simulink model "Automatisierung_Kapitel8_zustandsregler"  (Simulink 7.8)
settings: Solver=ode45  StartTime=0.0  StopTime=100  MaxStep=0.2  RelTol=1e-3
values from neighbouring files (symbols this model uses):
  Ac = [0,1,0,0;-1,-1,1,1;0,0,0,1;0.1,0.1,-0.2,-0.2]    [Automatisierung_Kapitel8.m]
  Bc = [bc,bvc]    [Automatisierung_Kapitel8.m]
  Cc = eye(4)    [Automatisierung_Kapitel8.m]
  Dc = [0,0;0,0;0,0;0,0]    [Automatisierung_Kapitel8.m]
  g = 1/((cc+dc*k)*inv(eye(4)-Ad-bd*k)*bd+dc)    [Automatisierung_Kapitel8.m]
  k = -acker(Ad,bd,pd)    [Automatisierung_Kapitel8.m]
  Ta = 2    [Automatisierung_Kapitel8.m]
libraries: simulink x1

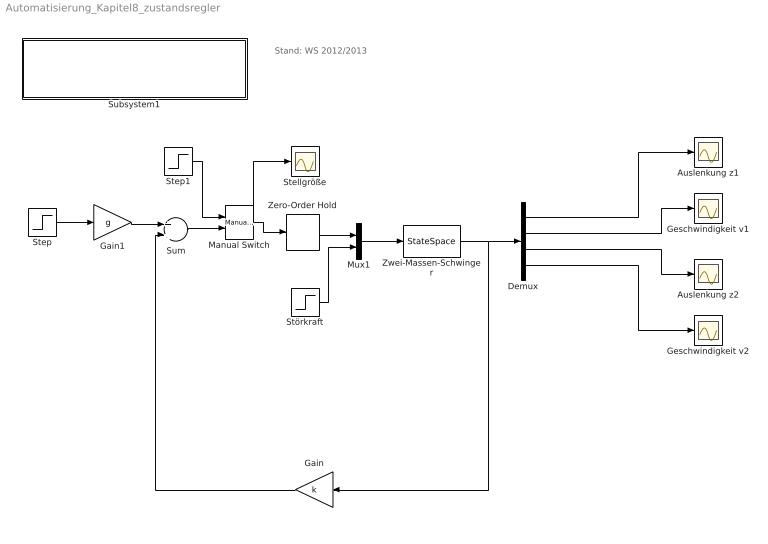
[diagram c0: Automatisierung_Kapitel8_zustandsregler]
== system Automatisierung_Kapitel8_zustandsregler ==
  note: Stand: WS 2012/2013
  Auslenkung z1 : Scope
  Auslenkung z2 : Scope
  Demux : Demux
  Gain : Gain  Gain=k  Multiplication=Matrix(K*u)  SampleTime=Ta
  Gain1 : Gain  Gain=g  SampleTime=Ta
  Geschwindigkeit v1 : Scope
  Geschwindigkeit v2 : Scope
  Manual Switch : simulink/Signal Routing/Manual Switch  sw=0  action=0  varsize=off
  Mux1 : Mux  Inputs=2
  Stellgröße : Scope
  Step : Step  Time=0  SampleTime=Ta
  Step1 : Step  Time=0  SampleTime=0
  Störkraft : Step  Time=20  SampleTime=Ta
  Subsystem1 : Subsystem
  Sum : Sum
  Zero-Order Hold : ZeroOrderHold  SampleTime=Ta
  Zwei-Massen-Schwinger : StateSpace  A=Ac  B=Bc  C=Cc  D=Dc  X0=[0,0,0,0]
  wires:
  Zwei-Massen-Schwinger/1 -> Demux/1, Gain/1
  Mux1/1 -> Zwei-Massen-Schwinger/1
  Störkraft/1 -> Mux1/2
  Demux/1 -> Auslenkung z1/1
  Demux/3 -> Auslenkung z2/1
  Step/1 -> Gain1/1
  Demux/2 -> Geschwindigkeit v1/1
  Demux/4 -> Geschwindigkeit v2/1
  Gain/1 -> Sum/2
  Gain1/1 -> Sum/1
  Sum/1 -> Manual Switch/2
  Manual Switch/1 -> Stellgröße/1, Zero-Order Hold/1
  Step1/1 -> Manual Switch/1
  Zero-Order Hold/1 -> Mux1/1

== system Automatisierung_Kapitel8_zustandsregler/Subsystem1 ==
